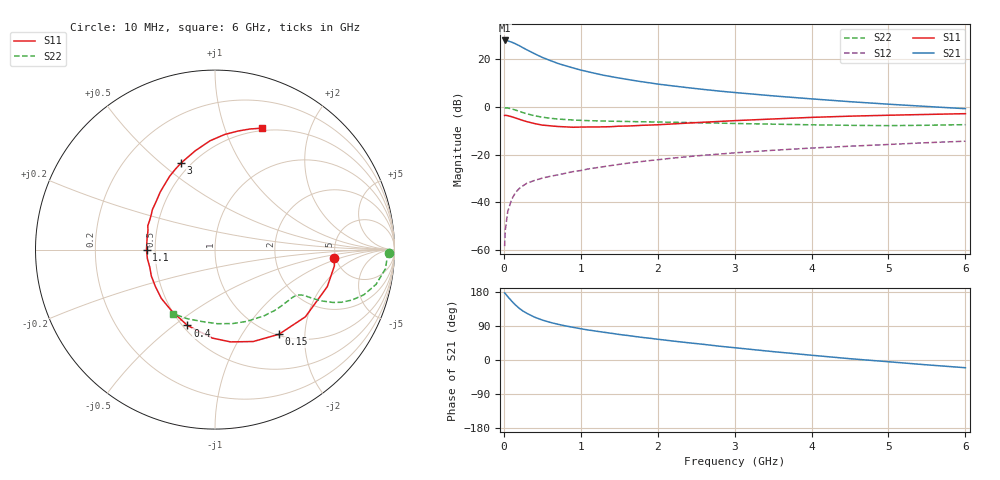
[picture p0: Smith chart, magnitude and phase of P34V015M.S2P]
! SIEMENS Small Signal Semiconductors
! BFP181
! Si NPN RF Bipolar Junction Transistor in SOT143
! VCE = 4 V  IC = 15 mA
! Common Emitter S-Parameters:  March  1996
# GHz  S  MA  R  50
!  f  S11  S21  S12  S22
! GHz  MAG  ANG  MAG  ANG  MAG  ANG  MAG  ANG
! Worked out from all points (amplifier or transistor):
!   36 points, 10 MHz to 6 GHz, reference 50 ohm
!   highest |S21| = 28.0 dB at 10 MHz (marker M1)
!   |S21| within 3 dB of that: start of sweep to 245 MHz
!   unconditionally stable (mu >= 1): 866 MHz to end of sweep
!   at 250 MHz: K = 0.45, MSG = 29.0 dB, |S12| = -33.0 dB
!   at 1.4 GHz: K = 1.16, MAG = 16.2 dB, |S12| = -24.5 dB
!   at 6 GHz: K = 1.01, MAG = 6.4 dB, |S12| = -14.3 dB
!   S11 on the Smith chart (normalised r, x): 10 MHz: 4.87, -0.77; 150 MHz: 1.02, -1.48; 400 MHz: 0.53, -0.56; 1.1 GHz: 0.45, -0.00; 3 GHz: 0.44, +0.59; 6 GHz: 0.47, +1.35
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0.01  0.6664 -3.8  25.01 177.1  0.0012 86.2  0.9686 -1.0
0.02  0.6713 -7.8  24.88 175.1  0.0027 83.7  0.961 -2.4
0.05  0.6587 -18.3  24.57 167.5  0.0063 84.4  0.9557 -6.4
0.1  0.6277 -36.6  23.05 155.9  0.0114 70.9  0.918 -12.2
0.15  0.5912 -52.9  21.35 145.4  0.0159 67.9  0.8666 -16.9
0.2  0.5547 -67.4  19.49 136.5  0.0195 63.1  0.8135 -20.2
0.25  0.5217 -80.4  17.52 129.0  0.0223 58.2  0.7636 -22.6
0.3  0.4932 -91.7  15.9 123.2  0.0252 56.9  0.7212 -24.1
0.4  0.4496 -110.0  13.15 113.0  0.0288 53.3  0.6564 -25.8
0.5  0.4178 -125.6  11.02 105.4  0.0322 52.4  0.6122 -26.5
0.6  0.4043 -137.7  9.528 99.4  0.0351 52.2  0.5822 -26.9
0.7  0.3904 -148.5  8.263 94.4  0.0376 52.2  0.5605 -27.2
0.9  0.3764 -165.0  6.629 86.3  0.0441 52.9  0.5345 -28.2
1.1  0.3816 -179.4  5.486 79.1  0.0503 53.0  0.5181 -29.6
1.5  0.3974 160.3  4.059 67.4  0.0626 53.1  0.5009 -33.5
1.8  0.4139 147.4  3.391 59.6  0.0721 52.3  0.4907 -37.5
2.2  0.4425 133.7  2.774 50.0  0.0849 50.3  0.479 -43.2
3  0.5183 111.4  2.021 32.4  0.1093 45.0  0.4519 -56.4
3.5  0.5619 101.2  1.716 22.1  0.1237 41.3  0.4374 -66.1
4.5  0.6437 85.2  1.296 3.4  0.1506 33.4  0.4131 -88.2
5.5  0.6998 73.8  1.028 -12.8  0.1785 26.0  0.4146 -111.6
6  0.7262 68.7  0.924 -20.4  0.1919 21.8  0.4272 -123.4
